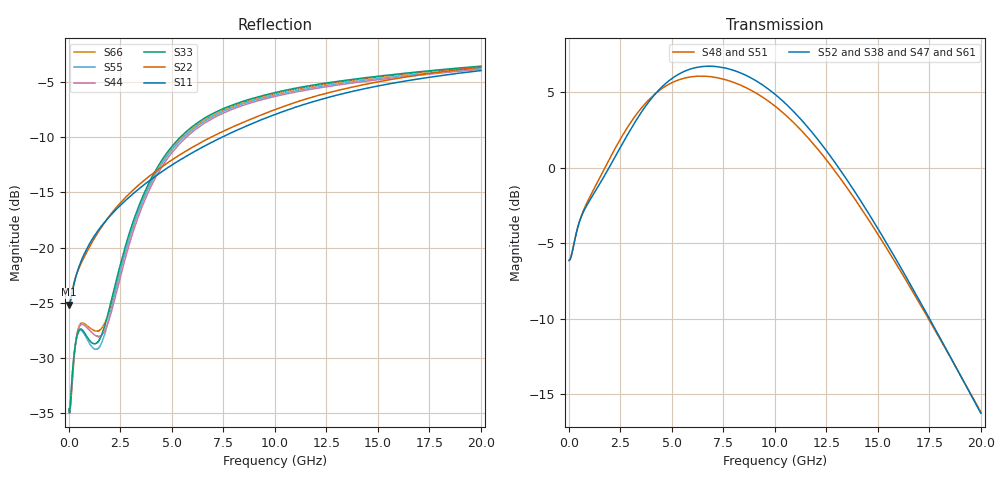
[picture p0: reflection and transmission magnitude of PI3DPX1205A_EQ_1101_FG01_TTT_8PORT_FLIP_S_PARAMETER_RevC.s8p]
! NPort=8 DATA=2000 NOISE=0 GROUPDELAY=0 COMPLEX_DATAFORMAT=POLAR
! NumOfBlock=1 NumOfParam=0
! .MODEL Smodel S TSTONEFILE=PI3DPX1205A_EQ_1101_FG01_TTT_8PORT_FLIP_S_PARAMETER_RevC.s8p TYPE=S
!  -- The above .MODEL line can be used for the S element in the netlist.
! The s parameter is extracted from the linear redriver, it is not bi-directional;
! only s(5,1)s(6,2)s(3,7)s(4,8) should be the insertion loss
!  Port definition:
!  Port1 = AIP
!  Port2 = AIN
!  Port3 = BOP
!  Port4 = BON
!  Port5 = AOP
!  Port6 = AON
!  Port7 = BIP
!  Port8 = BIN
# Hz S MA R  50
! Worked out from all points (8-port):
!   2000 points, 10 MHz to 20 GHz, reference 50 ohm
!   strongest paths, dB at 10 MHz, 5.01 GHz, 10.01 GHz, 15.01 GHz, 20 GHz:
!     S52: -6.1, 5.9, 4.9, -4.1, -16.3
!     S38: -6.1, 5.9, 4.8, -4.1, -16.3
!     S47: -6.1, 5.9, 4.9, -4.0, -16.2
!     S61: -6.1, 5.9, 4.9, -4.0, -16.2
!     S48: -6.1, 5.6, 4.1, -4.4, -16.2
!     S51: -6.1, 5.6, 4.1, -4.4, -16.2
!   lowest |S11| = -25.2 dB at 10 MHz (marker M1), VSWR 1.12, Z = 44.8 - j0.115 ohm
!   |S11| at or under -10 dB: start of sweep to 7.449 GHz
